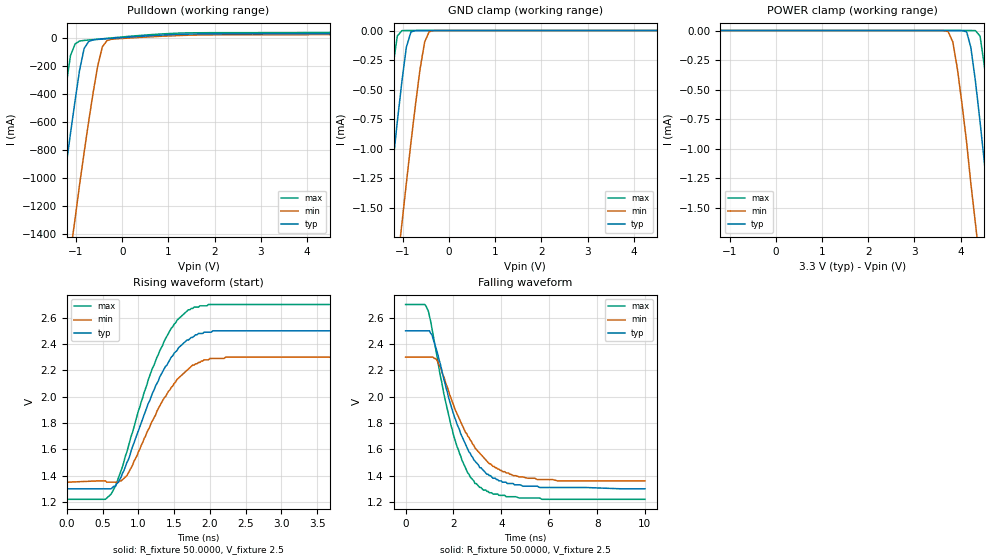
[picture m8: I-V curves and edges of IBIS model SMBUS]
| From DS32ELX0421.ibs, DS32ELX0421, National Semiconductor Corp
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|   Model SMBUS
[Model]  SMBUS
Model_type I/O_open_drain
Enable   Active-High
Vinl = 0V
Vinh = 2V
Vmeas = 1.4V
Vref = 2.5V
Rref = 50
C_comp   3.497pF   3.375pF   3.628pF
[Temperature Range]   25.0000   85.0000   -40.0000
[Voltage Range]   3.3000V   3.0000V   3.4650V
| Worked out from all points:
|   slope of the pulldown table from 0 to 0.495 V, typ, clamps not added: 44.3 ohm
|   GND clamp passes 1 mA (typ) near -1.18 V on its own axis
|   rising waveform, R_fixture 50.0000, V_fixture 2.5: 20-80 % time 547ps typ, 550ps min, 546ps max; typ from 1.3 V to 2.5 V
|   falling waveform, R_fixture 50.0000, V_fixture 2.5: 20-80 % time 1.37ns typ, 1.55ns min, 1.14ns max; typ from 2.5 V to 1.3 V
[GND_clamp]
|Voltage   I(typ)   I(min)   I(max)
-3.3V     -9.43mA    -10mA      -9.47mA
-1.62V    -2.67mA    -3.78mA    -1.96mA
-1.52V    -2.28mA    -3.41mA    -1.53mA
-1.42V    -1.89mA    -3.05mA    -1.11mA
-1.32V    -1.51mA    -2.7mA     -697uA
-1.12V    -771uA     -1.98mA    -46.7uA
-1.02V    -428uA     -1.63mA    -841nA
-924mV    -141uA     -1.29mA    -6.98nA
-825mV    -11.8uA    -948uA     -52pA
-627mV    -9.63nA    -325uA     -1.09pA
-429mV    -5.42pA    -9.52uA    -624fA
6.5V      13pA       12.4pA     13.3pA
|6.60E+00   1.32E-11   1.26E-11   1.35E-11
[POWER_clamp]
|Voltage   I(typ)   I(min)   I(max)
-3.2V     13pA       12.4pA     13.3pA
3.73V     -5.42pA    -9.52uA    -624fA
3.83V     -211pA     -96.3uA    -858fA
3.93V     -9.63nA    -325uA     -1.09pA
4.13V     -11.8uA    -948uA     -52pA
4.32V     -428uA     -1.63mA    -841nA
4.42V     -771uA     -1.98mA    -46.7uA
4.62V     -1.51mA    -2.7mA     -697uA
4.72V     -1.89mA    -3.05mA    -1.11mA
4.82V     -2.28mA    -3.41mA    -1.53mA
4.92V     -2.67mA    -3.78mA    -1.96mA
6.6V      -9.43mA    -10mA      -9.47mA
|-3.30E+00   1.32E-11   1.26E-11   1.35E-11
[Pulldown]
|Voltage   I(typ)   I(min)   I(max)
-3.3V     -6.71A     -7.29A     -6.59A
-1.62V    -1.96A     -2.79A     -1.44A
-1.42V    -1.44A     -2.28A     -879mA
-1.32V    -1.18A     -2.03A     -610mA
-1.12V    -683mA     -1.53A     -128mA
-1.02V    -449mA     -1.29A     -45.2mA
-924mV    -234mA     -1.05A     -24.2mA
-825mV    -77.9mA    -820mA     -19.9mA
-528mV    -12.8mA    -198mA     -11mA
-429mV    -10.4mA    -65.3mA    -8.06mA
-330mV    -8.04mA    -21.7mA    -5.06mA
6.5V      39.1mA     28.2mA     52.6mA
|6.60E+00   4.02E-02   2.89E-02   5.40E-02
[Ramp]
| variable   typ   min   max
dV/dt_r   718.160m/545.3p   567.475m/546.7p   888.620m/545.5p
dV/dt_f   716.85m/1.35n   567.073m/1.546n   888.227m/1.151n
R_load = 50.00
[Rising Waveform]
R_fixture= 50.0000
V_fixture= 2.5
V_fixture_min= 2.3
V_fixture_max= 2.7
|time   V(typ)   V(min)   V(max)
0s        1.3V       1.35V      1.22V
620ps     1.3V       1.35V      1.26V
720ps     1.35V      1.35V      1.38V
840ps     1.5V       1.4V       1.58V
1.08ns    1.86V      1.68V      2.03V
1.3ns     2.15V      1.93V      2.35V
1.54ns    2.35V      2.13V      2.58V
1.78ns    2.46V      2.24V      2.68V
2.22ns    2.5V       2.3V       2.7V
10ns      2.5V       2.3V       2.7V
[Falling Waveform]
R_fixture= 50.0000
V_fixture= 2.5
V_fixture_min= 2.3
V_fixture_max= 2.7
|time   V(typ)   V(min)   V(max)
0s        2.5V       2.3V       2.7V
800ps     2.5V       2.3V       2.7V
950ps     2.5V       2.3V       2.65V
1.3ns     2.35V      2.28V      2.32V
2ns       1.87V      1.94V      1.71V
2.6ns     1.6V       1.7V       1.42V
3.1ns     1.46V      1.57V      1.31V
3.65ns    1.38V      1.47V      1.26V
4.75ns    1.33V      1.39V      1.23V
10ns      1.3V       1.36V      1.22V
